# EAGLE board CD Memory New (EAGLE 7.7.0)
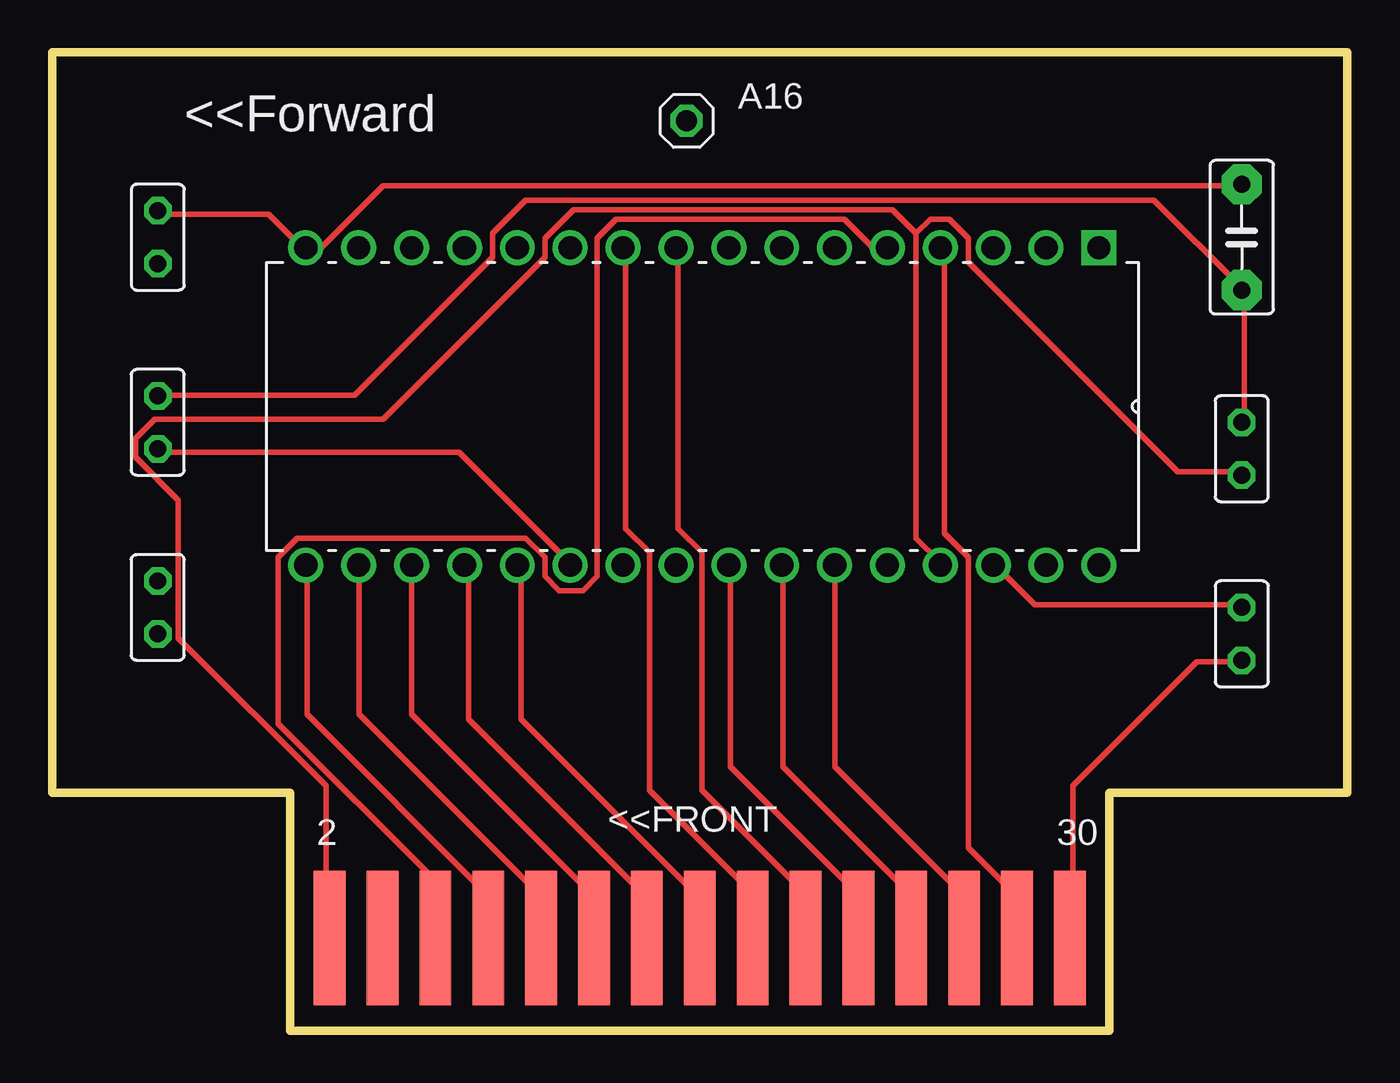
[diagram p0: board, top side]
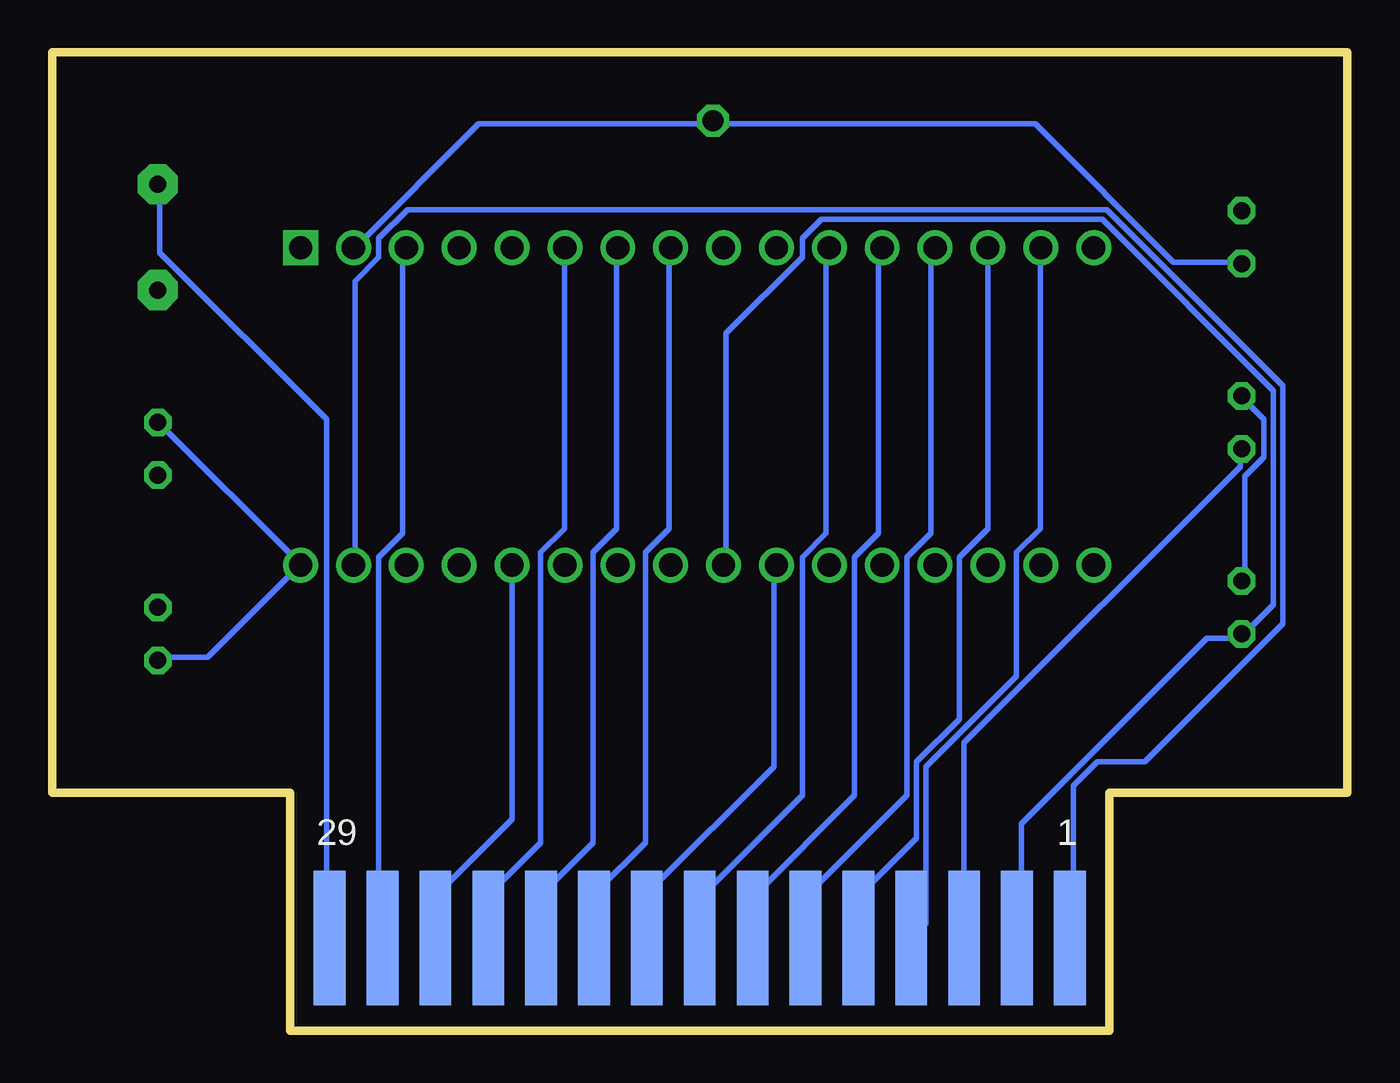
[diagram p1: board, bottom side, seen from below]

Size 62.23 x 46.99 mm. Coordinates in mm from the lower left corner, seen from the top.
Outline: 11.43,11.43 0,11.43 0,46.99 62.23,46.99 62.23,11.43 50.8,11.43 50.8,0 11.43,0 11.43,11.43
Copper layers (1*16): Top 0.035mm / dielectric 1.5mm / Bottom 0.035mm
Design rules "default": minimum track width 10mil, minimum drill 24mil, track to track 8mil, track to pad 8mil, pad to pad 8mil, via to via 8mil, smd to smd 8mil, copper to edge 40mil, drill to drill 8mil, minimum pad ring 10mil, minimum via ring 8mil, stop-mask expansion 4mil, vias tented up to drill 0mil, thermal gap 10mil

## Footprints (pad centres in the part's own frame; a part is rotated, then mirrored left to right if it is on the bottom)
1X01 = drill 1.016 octagon: 1 0,0
C050-030X075 = drill 0.813 pad 1.93 octagon: 1 -2.54,0; 2 2.54,0
DIP254P1524X393-32 = drill 1.118 pad 1.676 square: 1 -15.24,38.1 | drill 1.118 pad 1.676: 2 -15.24,35.56; 3 -15.24,33.02; 4 -15.24,30.48; 5 -15.24,27.94; 6 -15.24,25.4; 7 -15.24,22.86; 8 -15.24,20.32; 9 -15.24,17.78; 10 -15.24,15.24; 11 -15.24,12.7; 12 -15.24,10.16; 13 -15.24,7.62; 14 -15.24,5.08; 15 -15.24,2.54; 16 -15.24,0; 17 0,0; 18 0,2.54; 19 0,5.08; 20 0,7.62; 21 0,10.16; 22 0,12.7; 23 0,15.24; 24 0,17.78; 25 0,20.32; 26 0,22.86; 27 0,25.4; 28 0,27.94; 29 0,30.48; 30 0,33.02; 31 0,35.56; 32 0,38.1
V526-0 = drill 0.813 octagon: 1 -1.27,0; 2 1.27,0
J5CARD_NO_OUTLINE = smd 1.524 x 6.477 bottom: 1 -18.415,-5.715; 3 -15.875,-5.715; 5 -13.335,-5.715; 7 -10.795,-5.715; 9 -8.255,-5.715; 11 -5.715,-5.715; 13 -3.175,-5.715; 15 -0.635,-5.715; 17 1.905,-5.715; 19 4.445,-5.715; 21 6.985,-5.715; 23 9.525,-5.715; 25 12.065,-5.715; 27 14.605,-5.715; 29 17.145,-5.715 | smd 1.524 x 6.477: 2 -18.415,-5.715; 4 -15.875,-5.715; 6 -13.335,-5.715; 8 -10.795,-5.715; 10 -8.255,-5.715; 12 -5.715,-5.715; 14 -3.175,-5.715; 16 -0.635,-5.715; 18 1.905,-5.715; 20 4.445,-5.715; 22 6.985,-5.715; 24 9.525,-5.715; 26 12.065,-5.715; 28 14.605,-5.715; 30 17.145,-5.715

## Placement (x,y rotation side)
A16  [1X01]  30.48,43.69 0 top
C1  0.1uf  [C050-030X075]  57.15,38.1 270 top
IC1  AS6C1008-55PCN  [DIP254P1524X393-32]  12.19,22.35 270 top
R1  10K  [V526-0]  57.15,19.05 270 top
R2  10k  [V526-0]  57.15,27.94 90 top
R3  10K  [V526-0]  5.08,20.32 90 top
R4  10K  [V526-0]  5.08,29.21 90 top
R5  10k  [V526-0]  5.08,38.1 270 top
U$1  MEM_CARD_NO_OUTLINE  [J5CARD_NO_OUTLINE]  31.75,10.16 0 top

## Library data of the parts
A16 = pinhead
C1 R1-R5 = rcl
IC1 = SamacSys_Parts; DESCRIPTION: CMOS SRAM; HEIGHT: mm; MANUFACTURER_NAME: Alliance Memory; MANUFACTURER_PART_NUMBER: AS6C1008-55PCN; MOUSER_PART_NUMBER: 913-AS6C1008-55PCN; MOUSER_PRICE-STOCK: https://www.mouser.co.uk/ProductDetail/Alliance-Memory/AS6C1008-55PCN?qs=E5c5%252Bmu3i39qb4Qta5D2qg%3D%3D
U$1 = ADAM

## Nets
A0: IC1.12 U$1.13
A1: IC1.11 U$1.15
A2: IC1.10 U$1.18
A3: IC1.9 U$1.20
A4: IC1.8 U$1.19
A5: IC1.7 U$1.21
A6: IC1.6 U$1.23
A7: IC1.5 U$1.6
A8: IC1.27 U$1.26
A9: IC1.26 U$1.24
A10: IC1.23 U$1.17
A11: IC1.25 U$1.22
A12: IC1.4 U$1.28
A13: IC1.28 U$1.25
A14: IC1.3 U$1.27
A15: IC1.31 U$1.1
A16: A16.1 IC1.2 R5.2
CS: IC1.22 R4.1 U$1.5
D0: IC1.13 U$1.11
D1: IC1.14 U$1.9
D2: IC1.15 U$1.7
D3: IC1.17 U$1.8
D4: IC1.18 U$1.10
D5: IC1.19 U$1.12
D6: IC1.20 U$1.14
D7: IC1.21 U$1.16
N$1: IC1.30 R1.1
OE: IC1.24 R3.1 U$1.3
VCC: C1.2 IC1.32 R1.2 R2.2 R3.2 R4.2 U$1.30
VSS: C1.1 IC1.16 R5.1 U$1.29
WR: IC1.29 R2.1 U$1.2

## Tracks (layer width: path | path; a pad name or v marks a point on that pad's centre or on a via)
A0
  Bottom 0.254: IC1.12 22.53,37.59 22.53,23.88 23.67,22.73 23.67,11.3 28.47,6.5 28.47,4.45 U$1.13
A1
  Bottom 0.254: IC1.11 25.04,37.59 25.04,23.88 26.19,22.73 26.19,11.3 30.99,6.5 30.99,4.45 U$1.15
A2
  Top 0.254: IC1.10 27.56,37.59 27.56,24.11 28.7,22.96 28.7,11.53 33.5,6.73 33.5,4.45 U$1.18
A3
  Top 0.254: IC1.9 30.07,37.59 30.07,24.11 31.22,22.96 31.22,11.53 36.02,6.73 36.02,4.45 U$1.20
A4
  Bottom 0.254: IC1.8 32.59,37.59 32.59,24.11 33.73,22.96 33.73,9.02 36.02,6.73 36.02,4.45 U$1.19
A5
  Bottom 0.254: IC1.7 35.1,37.59 35.1,24.11 36.25,22.96 36.25,9.02 38.53,6.73 38.53,4.45 U$1.21
A6
  Bottom 0.254: U$1.23 41.28,6.5 38.76,9.02 38.76,22.96 37.62,24.11 37.62,37.59 IC1.6
A7
  Top 0.254: IC1.5 39.45,37.59 38.08,38.96 27.1,38.96 26.19,38.05 26.19,21.82 25.5,21.13 24.36,21.13 23.67,21.82 23.67,22.73 22.76,23.65 11.79,23.65 10.87,22.73 10.87,14.73 18.41,7.19 U$1.6
A8
  Top 0.254: IC1.27 37.62,22.28 37.62,12.68 43.79,6.5 43.79,4.45 U$1.26
A9
  Top 0.254: U$1.24 41.28,6.5 35.1,12.68 35.1,22.28 IC1.26
A10
  Bottom 0.254: IC1.23 27.56,22.28 27.56,12.68 33.5,6.73 33.5,4.45 U$1.17
A11
  Top 0.254: IC1.25 32.59,22.28 32.59,12.68 38.53,6.73 38.53,4.45 U$1.22
A12
  Top 0.254: IC1.4 42.88,37.59 42.88,23.88 44.02,22.73 44.02,8.79 46.3,6.5 46.3,4.45 U$1.28
A13
  Bottom 0.254: IC1.28 40.13,10.16 43.79,6.5 43.79,4.45 U$1.25
A14
  Bottom 0.254: IC1.3 45.39,37.59 45.39,23.88 46.53,22.73 46.53,4.45 U$1.27
A15
  Bottom 0.254: IC1.31 47.68,22.5 47.68,35.99 46.53,37.13 46.53,38.05 45.16,39.42 11.56,39.42 3.1,30.96 3.1,19.53 9.73,12.9 12.01,12.9 13.16,11.76 13.16,4.45 U$1.1
A16
  Bottom 0.254: R5.2 5.16,36.91 8.36,36.91 14.99,43.54 30.3,43.54 A16.1 30.53,43.54 41.73,43.54 47.68,37.59 IC1.2
CS
  Top 0.254: R4.1 5.16,27.76 19.56,27.76 24.82,22.5 IC1.22
  Bottom 0.254: U$1.5 18.41,13.82 5.16,27.08 5.16,27.76 R4.1
D0
  Bottom 0.254: IC1.13 20.02,37.59 20.02,23.88 21.16,22.73 21.16,11.3 25.96,6.5 25.96,4.45 U$1.11
D1
  Bottom 0.254: IC1.14 17.27,24.11 18.64,22.73 18.64,14.96 20.7,12.9 20.7,9.25 23.44,6.5 23.44,4.45 U$1.9
D2
  Bottom 0.254: IC1.15 14.76,37.59 14.76,24.11 15.9,22.96 15.9,17.02 20.24,12.68 20.24,5.13 20.93,4.45 U$1.7
D3
  Top 0.254: IC1.17 12.24,22.28 12.24,15.19 20.93,6.5 20.93,4.45 U$1.8
D4
  Top 0.254: IC1.18 14.76,22.28 14.76,15.19 23.44,6.5 23.44,4.45 U$1.10
D5
  Top 0.254: IC1.19 17.27,15.19 25.96,6.5 25.96,4.45 U$1.12
D6
  Top 0.254: IC1.20 20.02,22.28 20.02,14.96 28.47,6.5 28.47,4.45 U$1.14
D7
  Top 0.254: IC1.21 22.53,22.28 22.53,14.96 30.99,6.5 30.99,4.45 U$1.16
N$1
  Top 0.254: R1.1 57.05,20.45 47.22,20.45 45.39,22.28 IC1.30
OE
  Bottom 0.254: U$1.3 15.67,4.45 15.67,9.93 6.76,18.85 5.16,18.85 R3.1 4.93,19.07 3.56,20.45 3.56,30.73 11.79,38.96 25.27,38.96 26.19,38.05 26.19,37.13 29.84,33.48 29.84,22.5 IC1.24
VCC
  Top 0.254: U$1.30 49.05,4.45 49.05,11.76 54.99,17.7 57.05,17.7 R1.2 | R2.2 57.28,29.36 57.28,35.53 C1.2 57.05,35.76 52.93,39.88 22.76,39.88 21.16,38.28 21.16,37.13 14.53,30.5 5.16,30.5 R4.2
  Bottom 0.254: R1.2 57.05,17.93 54.76,17.93 50.42,22.28 IC1.32 50.42,22.5 57.05,29.13 R2.2 | R3.2 4.93,21.59 4.93,26.62 4.01,27.53 4.01,29.36 4.93,30.28 R4.2
VSS
  Top 0.254: R5.1 5.16,39.19 10.41,39.19 12.01,37.59 IC1.16 12.93,37.59 15.9,40.56 57.05,40.56 C1.1
  Bottom 0.254: C1.1 57.05,40.56 57.05,37.36 49.05,29.36 49.05,4.45 U$1.29
WR
  Top 0.254: 41.5,38.28 42.19,38.96 43.1,38.96 44.02,38.05 44.02,36.91 54.08,26.85 57.05,26.85 R2.1 | 41.5,38.28 41.5,23.65 42.65,22.5 IC1.29 | 41.5,38.28 40.36,39.42 25.04,39.42 23.67,38.05 23.67,37.13 15.9,29.36 4.93,29.36 4.01,28.45 4.01,27.53 6.07,25.48 6.07,18.85 13.16,11.76 13.16,4.45 U$1.2

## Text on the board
tNames: <<Forward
